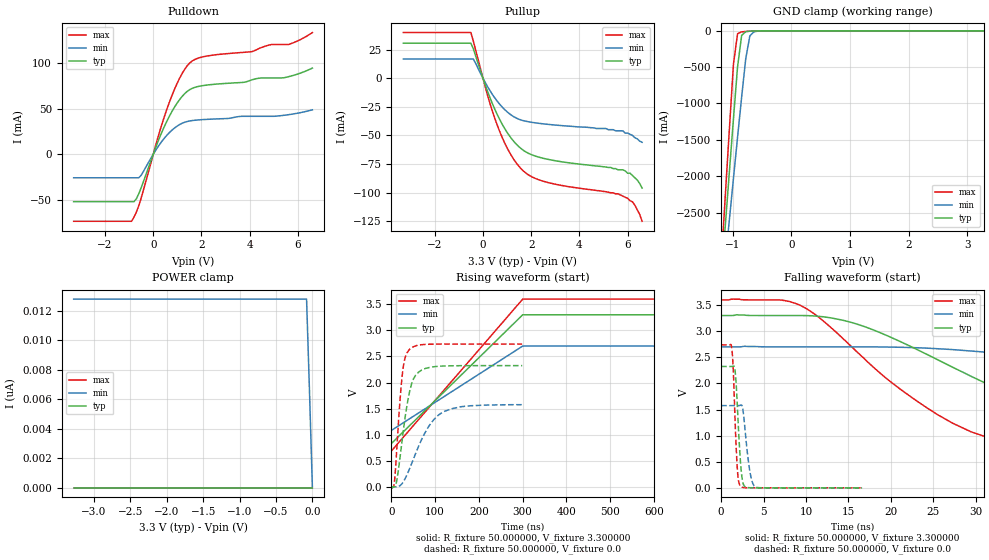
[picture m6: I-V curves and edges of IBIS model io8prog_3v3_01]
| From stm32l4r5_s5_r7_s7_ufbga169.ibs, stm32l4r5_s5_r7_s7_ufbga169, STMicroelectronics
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|   Model io8prog_3v3_01
[Model]  io8prog_3v3_01
Model_type I/O
Polarity   Non-Inverting
Enable   Active-Low
Vinl =   0.990000V
Vinh =   2.310000V
Vmeas =  1.650000V
Cref =   100.000000nF
Rref =   1.000000k
Vref =   3.300000V
C_comp   2.267200pF   2.233100pF   2.322300pF
[Temperature Range]   25.000000   0.125000k   -40.000000
[Pullup Reference]   3.300000V   2.700000V   3.600000V
[Pulldown Reference]   0.0V   0.0V   0.0V
[POWER Clamp Reference]   3.300000V   2.700000V   3.600000V
[GND Clamp Reference]   0.0V   0.0V   0.0V
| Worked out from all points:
|   slope of the pulldown table from 0 to 0.495 V, typ, clamps not added: 15.3 ohm
|   slope of the pullup table from 0 to 0.495 V, typ, clamps not added: 18.1 ohm
|   GND clamp passes 1 mA (typ) near -0.58 V on its own axis
|   rising waveform, R_fixture 50.000000, V_fixture 3.300000: 20-80 % time 180ns typ, 180ns min, 180ns max; typ from 0.831 V to 3.3 V
|   rising waveform, R_fixture 50.000000, V_fixture 0.0: 20-80 % time 24.3ns typ, 54.4ns min, 14.6ns max; typ from 0 V to 2.33 V
|   falling waveform, R_fixture 50.000000, V_fixture 3.300000: 20-80 % time 21ns typ, 41.5ns min, 13.6ns max; typ from 3.3 V to 0.831 V
|   falling waveform, R_fixture 50.000000, V_fixture 0.0: 20-80 % time 475ps typ, 656ps min, 393ps max; typ from 2.33 V to 0 V
[Pulldown]
|Voltage   I(typ)   I(min)   I(max)
-3.3V     -51.87mA   -25.68mA   -73.32mA
-900mV    -51.87mA   -25.68mA   -73.32mA
-700mV    -48.68mA   -25.68mA   -63.27mA
-500mV    -36.68mA   -22.92mA   -47.9mA
200mV     14.09mA    8.363mA    18.97mA
700mV     43.2mA     24.54mA    59.15mA
1.2V      63.38mA    34mA       88.53mA
1.6V      72.01mA    36.89mA    101.8mA
4.1V      81.58mA    41.61mA    112.4mA
4.9V      83.61mA    41.61mA    120.1mA
5.6V      84.89mA    43.33mA    120.1mA
6.6V      94.39mA    48.68mA    133.3mA
[Pullup]
|Voltage   I(typ)   I(min)   I(max)
-3.3V     30.51mA    16.73mA    39.79mA
-500mV    30.51mA    16.73mA    39.79mA
-400mV    25.73mA    16.73mA    32.44mA
200mV     -11.99mA   -7.69mA    -15.6mA
500mV     -27.53mA   -17.49mA   -35.6mA
1V        -47.29mA   -29.38mA   -60.81mA
1.5V      -60.05mA   -35.95mA   -77.15mA
1.9V      -65.77mA   -38.13mA   -84.64mA
2.6V      -70.47mA   -40.14mA   -90.6mA
5.6V      -80mA      -46mA      -101mA
6.2V      -85mA      -50mA      -108mA
6.6V      -96mA      -56mA      -125mA
[GND_clamp]
|Voltage   I(typ)   I(min)   I(max)
-3.3V     -9.456A    -9.706A    -9.779A
-1.2V     -3.441A    -3.76A     -3.218A
-1.13V    -2.694A    -3.182A    -2.288A
-1.06V    -1.951A    -2.607A    -1.365A
-990mV    -1.216A    -2.035A    -464.9mA
-920mV    -500mA     -1.468A    -40.15mA
-850mV    -63.51mA   -913mA     -13.79mA
-780mV    -11.84mA   -384.3mA   -8.858mA
-710mV    -4.78mA    -70.26mA   -5.228mA
-640mV    -2.25mA    -14.29mA   -2.447mA
-430mV    -27.1uA    -149uA     -11.19uA
3.28V     0A         0A         0A
[POWER_clamp]
|Voltage   I(typ)   I(min)   I(max)
-3.28V    0A         12.77nA    0A
-80mV     0A         12.77nA    0A
-40mV     0A         6.549nA    0A
0V        0A         0A         0A
[Ramp]
| variable   typ   min   max
dV/dt_r  1.39476/24.30683n   0.94506/54.41207n   1.64316/14.55319n
dV/dt_f  1.48126/21.06482n   0.97098/44.57739n   1.74767/13.63828n
R_load = 50.000000
[Rising Waveform]
R_fixture= 50.000000
V_fixture= 3.300000
V_fixture_min= 2.700000
V_fixture_max= 3.600000
|time   V(typ)   V(min)   V(max)
0s        831.2mV    1.082V     687.2mV
300.3ns   3.3V       2.7V       3.6V
600.6ns   3.3V       2.7V       3.6V
29.73us   3.3V       2.7V       3.6V
[Rising Waveform]
R_fixture= 50.000000
V_fixture= 0.0
V_fixture_min= 0.0
V_fixture_max= 0.0
|time   V(typ)   V(min)   V(max)
0s        2.592nV    41.12nV    2.445nV
7.207ns   2.235mV    -150.5uV   116.2mV
12.61ns   138.2mV    1.133mV    764.7mV
19.82ns   570.6mV    23mV       1.676V
27.03ns   1.062V     92.16mV    2.291V
39.64ns   1.743V     309.4mV    2.62V
61.86ns   2.198V     771.6mV    2.716V
87.09ns   2.289V     1.18V      2.735V
118.9ns   2.317V     1.439V     2.738V
299.1ns   2.325V     1.575V     2.739V
[Falling Waveform]
R_fixture= 50.000000
V_fixture= 3.300000
V_fixture_min= 2.700000
V_fixture_max= 3.600000
|time   V(typ)   V(min)   V(max)
0s        3.3V       2.7V       3.6V
9.309ns   3.3V       2.7V       3.497V
15.92ns   3.141V     2.7V       2.62V
25.53ns   2.453V     2.664V     1.402V
29.73ns   2.116V     2.617V     1.059V
35.14ns   1.728V     2.529V     872.5mV
45.65ns   1.184V     2.294V     770mV
56.76ns   995.6mV    2.009V     727.7mV
91.89ns   863.6mV    1.303V     693.4mV
149.5ns   831.2mV    1.082V     687.2mV
[Falling Waveform]
R_fixture= 50.000000
V_fixture= 0.0
V_fixture_min= 0.0
V_fixture_max= 0.0
|time   V(typ)   V(min)   V(max)
0s        2.325V     1.575V     2.739V
1.235ns   2.325V     1.575V     2.705V
1.435ns   2.33V      1.575V     2.254V
1.702ns   2.15V      1.575V     1.059V
1.969ns   1.384V     1.575V     246.7mV
2.302ns   455.6mV    1.584V     27.2mV
2.703ns   43.1mV     1.314V     4.228mV
3.403ns   2.827mV    303.3mV    1.778mV
4.037ns   1.379mV    17.38mV    1.399mV
16.62ns   2.592nV    41.12nV    2.445nV
